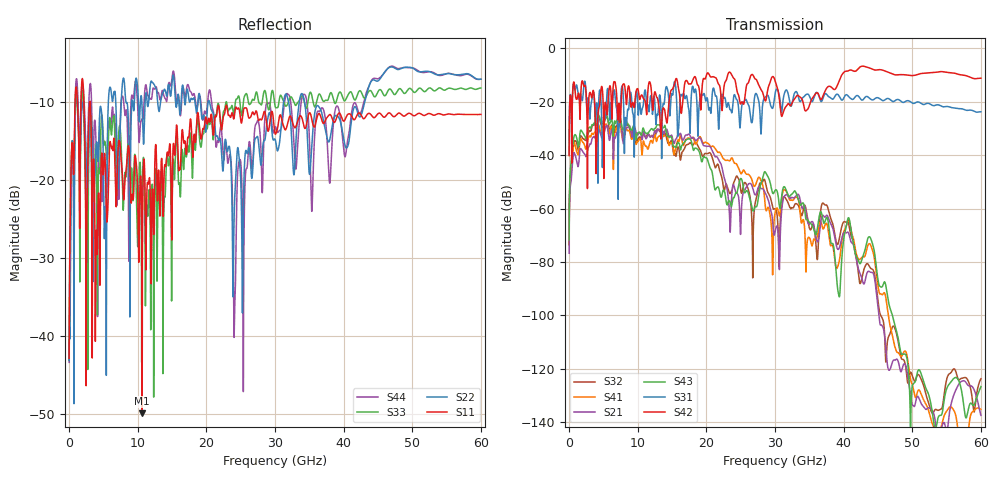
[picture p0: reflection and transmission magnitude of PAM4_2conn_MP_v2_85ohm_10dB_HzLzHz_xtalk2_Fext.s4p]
! Info: Touchstone file created by Circ.  Input file=FAB50GbE_2conn_Midplane_Examax_Topo2_v2_85ohm_10dB_HzLzHz.circ
# Hz S RI R 50
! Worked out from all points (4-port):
!   6000 points, 10 MHz to 60 GHz, reference 50 ohm
!   strongest paths, dB at 10 MHz, 15.01 GHz, 30.01 GHz, 45.01 GHz, 60 GHz:
!     S42: -40.1, -15.4, -12.0, -8.0, -11.2
!     S31: -39.8, -17.1, -17.1, -18.5, -23.7
!     S43: -71.7, -34.1, -53.2, -86.6, -126.6
!     S21: -76.7, -32.9, -68.7, -97.2, -137.4
!     S41: -73.4, -34.9, -61.6, -88.9, -135.1
!     S32: -73.4, -35.5, -60.1, -94.5, -123.7
!   lowest |S11| = -49.9 dB at 10.65 GHz (marker M1), VSWR 1.01, Z = 49.8 - j0.223 ohm
!   |S11| at or under -10 dB: start of sweep to 880.2 MHz; 2.164 GHz to 3.001 GHz (837.2 MHz wide, 32.4 % of centre); 3.082 GHz to end of sweep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
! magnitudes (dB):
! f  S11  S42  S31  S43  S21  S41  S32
! 10 MHz  -42.9  -40.1  -39.8  -71.7  -76.7  -73.4  -73.4
! 1.11 GHz  -8.3  -19.1  -13.7  -33.5  -42.1  -38.6  -35.4
! 10.65 GHz  -49.9  -17.6  -22.7  -31.4  -34.1  -39.9  -33.3
! 20.53 GHz  -12.5  -10.4  -22.3  -44.6  -36.7  -36.5  -39.1
! 24.12 GHz  -11.5  -11.5  -17.3  -55.3  -52.4  -43.0  -49.6
! 39.02 GHz  -11.9  -14.2  -17.1  -87.2  -74.6  -82.4  -73.2
! 60 GHz  -11.5  -11.2  -23.7  -126.6  -137.4  -135.1  -123.7
